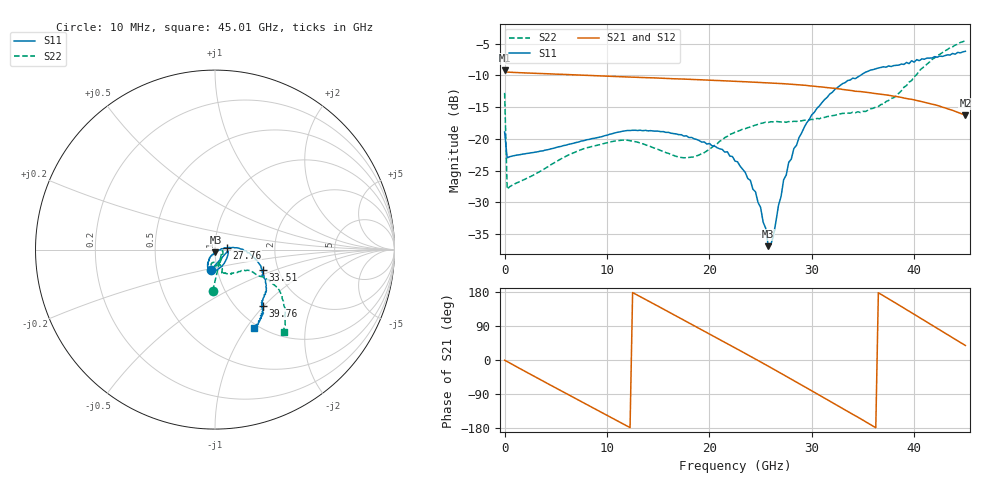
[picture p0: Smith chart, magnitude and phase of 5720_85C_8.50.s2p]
! Device:  ADRF5720
! Description: 0.5dB LSB GaAs MMIC 6-bit Digital Attenuator
! Frequency:  0.000009 -  40 GHz
! Ports:
!	RF1	= Port 1
!	RF2	= Port 2
! Vdd:  3.3 Volt
! Vss:  -3.3 Volt
! Control:  0/3.3 Volt
! State:  8.50 dB attenuation
! Data:  The device was measured using G-S-G Probes on a matrix board.
!  Data was collected using an calibrated 4 port network analyzer.
!  The reference plane for this measurement is at the launchers.
! Note:  Analog Devices supplies this data as a sample of measured data
!  for this product.  Your particular data for this product may vary.
!  Data was taken at 85 degrees C.
!  Analog Devices reserves the right to change this data at anytime.
# GHZ S DB R 45.0
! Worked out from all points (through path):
!   181 points, 10 MHz to 45.01 GHz, reference 45 ohm
!   highest |S21| = -9.16 dB at 10 MHz (marker M1); lowest = -16.3 dB at 45.01 GHz (marker M2)
!   group delay of S21, straight-line fit = 41.7 ps
!   lowest |S11| = -36.9 dB at 25.76 GHz (marker M3), VSWR 1.03, Z = 45.2 - j1.27 ohm
!   |S11| at or under -10 dB: start of sweep to 34.75 GHz
!   |S22| runs from -27.9 to -4.5 dB; largest |S21 - S12| = 0.0016
!   S11 on the Smith chart (normalised r, x): 10 MHz: 0.94, -0.21; 27.76 GHz: 1.14, +0.02; 33.51 GHz: 1.66, -0.41; 39.76 GHz: 1.31, -0.99; 45.01 GHz: 0.95, -1.09
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0.01  -18.91 -100.6  -9.16 -0.7  -9.15 -0.7  -12.75 -93.1
0.26  -22.99 -8.0  -9.46 -4.0  -9.46 -4.0  -27.92 -12.1
4.26  -21.70 -39.0  -9.74 -62.9  -9.72 -62.9  -24.37 -51.6
7.76  -20.29 -62.6  -9.96 -113.5  -9.95 -113.5  -21.55 -76.6
11.51  -18.80 -85.5  -10.21 -167.6  -10.19 -167.5  -20.20 -96.7
15.26  -18.86 -104.5  -10.42 138.1  -10.41 138.3  -21.84 -104.5
19.01  -20.26 -114.9  -10.67 83.5  -10.65 83.7  -22.55 -79.6
22.76  -23.62 -119.2  -10.94 28.4  -10.92 28.6  -18.80 -69.7
24.51  -28.34 -117.9  -11.07 2.4  -11.05 2.6  -17.83 -72.6
25.51  -34.10 -88.8  -11.14 -12.6  -11.12 -12.3  -17.36 -73.9
25.76  -36.92 -78.9  -11.16 -16.3  -11.15 -16.1  -17.41 -73.4
26.26  -35.34 -23.2  -11.20 -23.9  -11.19 -23.7  -17.31 -73.2
27.26  -26.43 6.3  -11.30 -39.1  -11.29 -38.9  -17.31 -72.8
27.76  -23.69 8.6  -11.35 -46.8  -11.34 -46.5  -17.27 -72.3
28.76  -19.79 6.7  -11.48 -62.0  -11.47 -61.7  -17.17 -70.7
30.26  -15.80 -2.4  -11.70 -85.2  -11.69 -84.9  -16.98 -67.1
33.51  -10.80 -23.4  -12.30 -135.6  -12.28 -135.3  -15.94 -58.3
35.76  -9.14 -35.1  -12.74 -170.8  -12.73 -170.5  -15.25 -49.2
37.76  -8.59 -42.4  -13.20 157.3  -13.18 157.7  -13.64 -34.3
39.76  -7.68 -49.5  -13.76 124.7  -13.74 125.0  -10.80 -30.9
42.26  -7.12 -54.1  -14.72 83.4  -14.70 83.9  -6.87 -34.6
45.01  -6.19 -63.5  -16.28 38.3  -16.25 38.7  -4.48 -50.2
